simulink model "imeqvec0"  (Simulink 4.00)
settings: Solver=ode45  StartTime=0.0  StopTime=1  MaxStep=1e-3  RelTol=1e-3
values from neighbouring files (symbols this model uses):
  H = 0.60    (= 0.6)    [IMabc2.m]    (also in IMcur0.m = 0.3; imdef0vec.m = 0.3; imdef1vec.m = 0.3; imdef2vec.m = 0.3)
  ic = [fs0 fr0]    [imdef0vec.m]    (also in imdef1vec.m; imdef2vec.m = F; imic2.m = [phids phiqs phidr phiqr n0]'; imic3.m = [phids phiqs phidr phiqr n0]')
  Lm = eval(get(hLm,'String'))    [im3d.m]    (also in IMabc2.m = 4.5; imabcparam.m = 0.0847; IMabcrun0.m = 0.0847; IMabcrun1.m = 0.0847)
  Lrl = eval(get(hLr,'String'))    [im3d.m]    (also in IMabc2.m = 0.1; imabcparam.m = 0.0025; IMabcrun0.m = 0.0025; IMabcrun1.m = 0.0025)
  Lsl = eval(get(hLs,'String'))    [im3d.m]    (also in IMabc2.m = 0.1; imabcparam.m = 0.0025; IMabcrun0.m = 0.0025; IMabcrun1.m = 0.0025)
  n0 = 0.98    [imdef0vec.m]    (also in imdef1vec.m = 0.978; imdef2vec.m; imdefrotflux.m; imdefSIvec1.m = 0.95)
  Rr = input('Rotor resistance)[default = 2] =')    [Actac.m]    (also in im1phase.m = 0.3; im3d.m = eval(get(hRr,'String')); IMabc2.m = 0.02; imabcparam.m = 0.408)
  Rs = eval(get(hRs,'String'))    [im3d.m]    (also in IMabc2.m = 0.01; imabcparam.m = 0.531; IMabcrun0.m = 0.531; IMabcrun1.m = 0.531)
  Tl0 = Is*conj(Is)*Req    [imdef0vec.m]    (also in imdef1vec.m; imdef2vec.m = Lm*(I(2)*I(3)-I(1)*I(4)); imdefrotflux.m; imdefSIvec1.m = Te0/To)
  vs = 1.0    (= 1)    [imdef0vec.m]    (also in imdef1vec.m; imdef2vec.m; imdefrotflux.m; imdefSIvec1.m)
  wk = ws    (= 1)    [imdef0vec.m]    (also in imdef1vec.m; imdef2vec.m; imdefrotflux.m; imdefSIvec1.m)
  wo = 2*pi*freq0    [calc0.m]    (also in IMabc2.m = 376.991118431; imabcparam.m = 376.991118431; IMabcrun0.m = 376.991118431; IMabcrun1.m = 376.991118431)
libraries: simulink3 x1

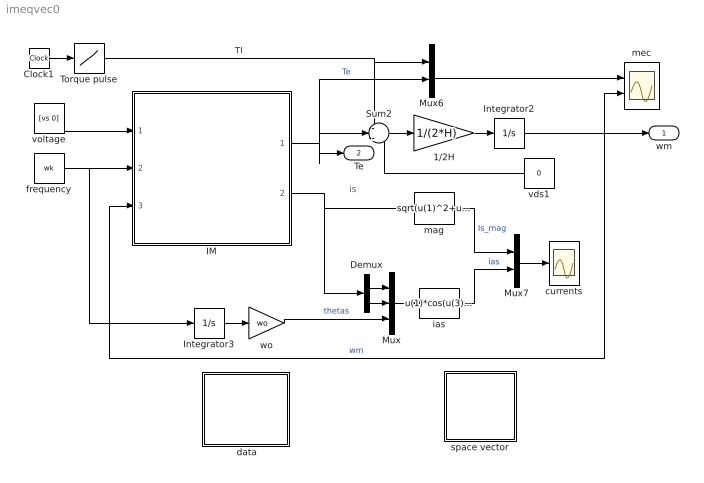
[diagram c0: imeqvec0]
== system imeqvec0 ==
  note: is
  " data" : Subsystem
  1/2H : Gain  Gain=1/(2*H)  Multiplication=Element-wise(K.*u)  SaturateOnIntegerOverflow=on
  Clock1 : Clock
  Demux : Demux  Outputs=2  BusSelectionMode=off
  IM : Subsystem
  Integrator2 : Integrator  ExternalReset=none  InitialConditionSource=internal  InitialCondition=n0  LimitOutput=off  UpperSaturationLimit=inf  LowerSaturationLimit=-inf  ShowSaturationPort=off  ShowStatePort=off  AbsoluteTolerance=auto
  Integrator3 : Integrator  ExternalReset=none  InitialConditionSource=internal  InitialCondition=0  LimitOutput=off  UpperSaturationLimit=inf  LowerSaturationLimit=-inf  ShowSaturationPort=off  ShowStatePort=off  AbsoluteTolerance=auto
  Mux : Mux  Inputs=3
  Mux6 : Mux  Inputs=2
  Mux7 : Mux  Inputs=2
  Sum2 : Sum  Inputs=-+-  SaturateOnIntegerOverflow=on
  Torque pulse : Lookup  InputValues=[0 0.1 0.1 0.5 0.5 2]  OutputValues="[Tl0 Tl0  0 0 0.5 0.5]"
  currents : Scope
  frequency : Constant  Value=wk
  ias : Fcn  Expr=u(1)*cos(u(3))-u(2)*sin(u(3))
  mag : Fcn  Expr=sqrt(u(1)^2+u(2)^2)
  mec : Scope  NumInputPorts=2
  space vector : Subsystem
  vds1 : Constant  Orientation=left  Value=0
  voltage : Constant  Value=[vs 0]
  wo : Gain  Gain=wo  Multiplication=Element-wise(K.*u)  SaturateOnIntegerOverflow=on
  wm : Outport  Port=1
  Te : Outport  Port=2
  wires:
  voltage/1 -> IM/1(vs)
  frequency/1 -> Integrator3/1, IM/2(Iwk)
  Demux/1 -> Mux/1
  Demux/2 -> Mux/2
  Mux/1 -> ias/1
  ias/1 -> Mux7/2  "ias"
  mag/1 -> Mux7/1  "Is_mag"
  Mux7/1 -> currents/1
  IM/2(is) -> mag/1, Demux/1
  Sum2/1 -> 1/2H/1
  1/2H/1 -> Integrator2/1
  Clock1/1 -> Torque pulse/1
  Mux6/1 -> mec/1
  IM/1(Te) -> Sum2/2, Mux6/2, Te/1  "Te"
  Torque pulse/1 -> Mux6/1, Sum2/1  "Tl"
  vds1/1 -> Sum2/3
  Integrator3/1 -> wo/1
  wo/1 -> Mux/3  "thetas"
  Integrator2/1 -> mec/2, IM/3(wm), wm/1  "wm"

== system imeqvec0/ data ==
  note: This demo simulates the running of an induction motor in steady-state when a sudden input change is effected: a)torque step changes at constant voltage excitation b) voltage input sag at constant frequency and load torque c)simultaneous step changes in voltage magnitude and frequency
  note: Double click the block to enter the machine parameters and initial conditions and then run the simulation

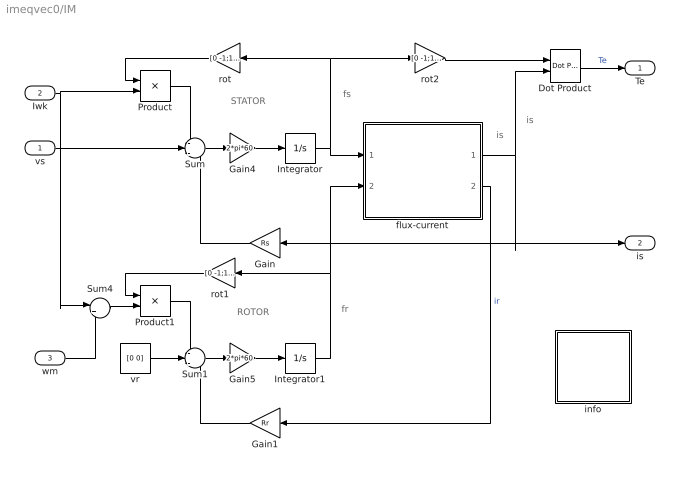
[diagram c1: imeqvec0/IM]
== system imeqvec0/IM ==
  note: ROTOR
  note: STATOR
  note: fs
  note: fr
  note: is
  note: is
  vs : Inport  Port=1
  Iwk : Inport  Port=2
  wm : Inport  Port=3
  Dot Product : simulink3/Math/Dot Product
  Gain : Gain  Orientation=left  Gain=Rs  Multiplication=Element-wise(K.*u)  SaturateOnIntegerOverflow=on
  Gain1 : Gain  Orientation=left  Gain=Rr  Multiplication=Element-wise(K.*u)  SaturateOnIntegerOverflow=on
  Gain4 : Gain  Gain=2*pi*60  Multiplication=Element-wise(K.*u)  SaturateOnIntegerOverflow=on
  Gain5 : Gain  Gain=2*pi*60  Multiplication=Element-wise(K.*u)  SaturateOnIntegerOverflow=on
  Integrator : Integrator  ExternalReset=none  InitialConditionSource=internal  InitialCondition=[ic(1) ic(2)]  LimitOutput=off  UpperSaturationLimit=inf  LowerSaturationLimit=-inf  ShowSaturationPort=off  ShowStatePort=off  AbsoluteTolerance=auto
  Integrator1 : Integrator  ExternalReset=none  InitialConditionSource=internal  InitialCondition=[ic(3) ic(4)]  LimitOutput=off  UpperSaturationLimit=inf  LowerSaturationLimit=-inf  ShowSaturationPort=off  ShowStatePort=off  AbsoluteTolerance=auto
  Product : Product  Inputs=2  Multiplication=Element-wise(.*)  SaturateOnIntegerOverflow=on
  Product1 : Product  Inputs=2  Multiplication=Element-wise(.*)  SaturateOnIntegerOverflow=on
  Sum : Sum  Inputs=-+-  SaturateOnIntegerOverflow=on
  Sum1 : Sum  Inputs=-+-  SaturateOnIntegerOverflow=on
  Sum4 : Sum  Inputs=|+-  SaturateOnIntegerOverflow=on
  flux-current : Subsystem
  info : Subsystem
  rot : Gain  Orientation=left  Gain=[0 -1;1 0]  Multiplication=Matrix(K*u)  SaturateOnIntegerOverflow=on
  rot1 : Gain  Orientation=left  Gain=[0 -1;1 0]  Multiplication=Matrix(K*u)  SaturateOnIntegerOverflow=on
  rot2 : Gain  Gain=[0 -1;1 0]  Multiplication=Matrix(K*u)  SaturateOnIntegerOverflow=on
  vr : Constant  Value=[0 0]
  Te : Outport  Port=1
  is : Outport  Port=2
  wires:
  Gain/1 -> Sum/3
  vr/1 -> Sum1/2
  Gain1/1 -> Sum1/3
  flux-current/2(ir) -> Gain1/1  "ir"
  Integrator/1 -> flux-current/1(fs), rot/1, rot2/1
  Integrator1/1 -> flux-current/2(fr), rot1/1
  Product1/1 -> Sum1/1
  rot1/1 -> Product1/1
  Product/1 -> Sum/1
  rot/1 -> Product/1
  rot2/1 -> Dot Product/1
  Sum4/1 -> Product1/2
  Sum/1 -> Gain4/1
  Gain4/1 -> Integrator/1
  Sum1/1 -> Gain5/1
  Gain5/1 -> Integrator1/1
  flux-current/1(is) -> Dot Product/2, Gain/1, is/1
  Dot Product/1 -> Te/1  "Te"
  vs/1 -> Sum/2
  Iwk/1 -> Product/2, Sum4/1
  wm/1 -> Sum4/2

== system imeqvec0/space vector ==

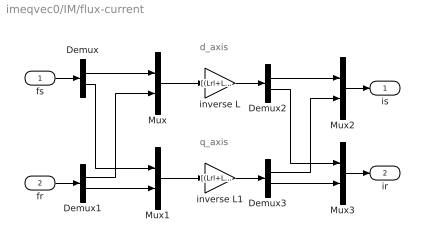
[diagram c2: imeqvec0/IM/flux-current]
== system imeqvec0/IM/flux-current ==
  note: d_axis
  note: q_axis
  fs : Inport  Port=1
  fr : Inport  Port=2
  Demux{,1..3} (4 alike) : Demux  Outputs=2  BusSelectionMode=off
  Mux{,1..3} (4 alike) : Mux  Inputs=2
  inverse L : Gain  Gain=[(Lrl+Lm) -Lm;-Lm (Lsl+Lm)]/(Lsl*Lrl+Lsl*Lm+Lrl*Lm)  Multiplication=Matrix(K*u)  SaturateOnIntegerOverflow=on
  inverse L1 : Gain  Gain=[(Lrl+Lm) -Lm;-Lm (Lsl+Lm)]/(Lsl*Lrl+Lsl*Lm+Lrl*Lm)  Multiplication=Matrix(K*u)  SaturateOnIntegerOverflow=on
  is : Outport  Port=1
  ir : Outport  Port=2
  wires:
  Demux/1 -> Mux/1
  Mux/1 -> inverse L/1
  inverse L/1 -> Demux2/1
  Demux2/1 -> Mux2/1
  fs/1 -> Demux/1
  Mux2/1 -> is/1
  Demux1/1 -> Mux/2
  Demux1/2 -> Mux1/2
  Demux/2 -> Mux1/1
  Mux1/1 -> inverse L1/1
  inverse L1/1 -> Demux3/1
  Demux3/2 -> Mux3/2
  Demux2/2 -> Mux3/1
  Demux3/1 -> Mux2/2
  Mux3/1 -> ir/1
  fr/1 -> Demux1/1

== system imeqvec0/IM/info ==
  note: Mathematical model of the induction machine. State vector formulation in an arbitrary dq common reference frame. Per unit description.
  note: Electrical system equations: vs = Rs.is + 1/wo.(dfs/dt) + j.wk.fs vr = Rr.ir + 1/wo.(dfr/dt) + j.(wk - wm).fr where the variables i, v, and f are 2-dimensional space vectors; for instance is = [ids iqs] and so forth and j represents a 90o space rotator namely j = [0 -1;1 0] The flux linkage current relations are: fds = (Lm + Lsl).ids + Lm.idr fdr = Lm.ids + (Lm + Lrl).idr (D_axis) fqs = (Lm + Lsl).iqs + Lm.iqr fqr = Lm.iqs + (Lm + Lrl).iqr (Q_axis) Mechanical system equations: Te = 2H.dwm/dt + Bm.wm + Tl where Te = fs (cross) is = j.fs (dot) is
